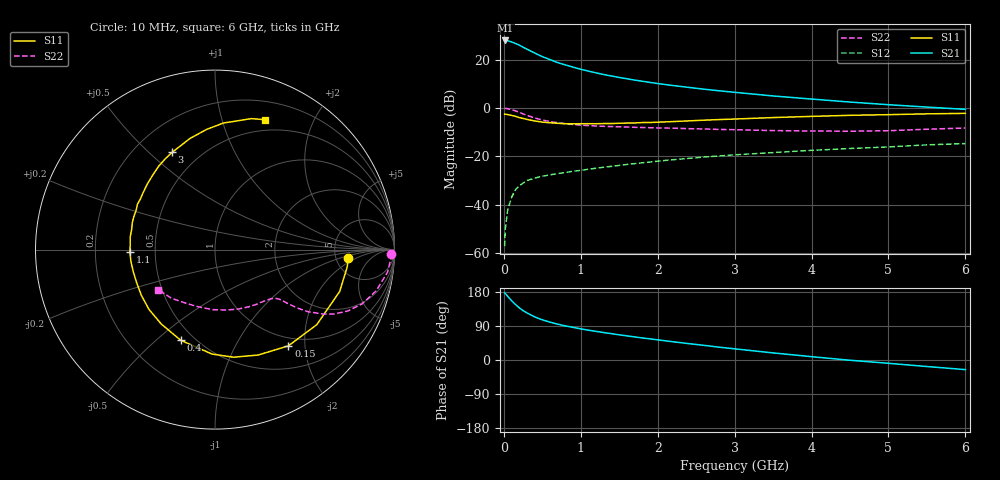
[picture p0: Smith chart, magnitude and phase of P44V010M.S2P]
! SIEMENS Small Signal Semiconductors
! BFP182
! Si NPN RF Bipolar Junction Transistor in SOT143
! VCE = 4 V  IC = 10 mA
! Common Emitter S-Parameters:  March  1996
# GHz  S  MA  R  50
!  f  S11  S21  S12  S22
! GHz  MAG  ANG  MAG  ANG  MAG  ANG  MAG  ANG
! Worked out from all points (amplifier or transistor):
!   36 points, 10 MHz to 6 GHz, reference 50 ohm
!   highest |S21| = 27.9 dB at 20 MHz (marker M1)
!   |S21| within 3 dB of that: start of sweep to 263.1 MHz
!   unconditionally stable (mu >= 1): 1.182 GHz to 5.382 GHz
!   at 250 MHz: K = 0.33, MSG = 28.1 dB, |S12| = -31.0 dB
!   at 1.4 GHz: K = 1.07, MAG = 17.1 dB, |S12| = -24.1 dB
!   at 6 GHz: K = 0.94, MSG = 7.1 dB, |S12| = -14.7 dB
!   lowest NFmin = 1.50 dB at 450 MHz
!   S11 on the Smith chart (normalised r, x): 10 MHz: 6.51, -1.40; 150 MHz: 0.86, -1.68; 400 MHz: 0.42, -0.60; 1.1 GHz: 0.36, -0.01; 3 GHz: 0.36, +0.59; 6 GHz: 0.38, +1.38
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0.01  0.7442 -3.7  24.84 177.5  0.0014 91.8  0.9828 -1.4
0.02  0.743 -7.5  24.86 175.4  0.0033 84.0  0.9813 -2.9
0.05  0.7327 -18.6  24.54 168.0  0.0078 83.6  0.9692 -7.5
0.1  0.7047 -36.4  23.18 156.8  0.0142 71.0  0.9265 -14.4
0.15  0.6743 -52.7  21.58 146.7  0.0204 65.5  0.8743 -20.2
0.2  0.6348 -67.7  19.93 137.7  0.0247 60.7  0.8151 -24.8
0.25  0.6084 -80.2  18.04 130.3  0.0281 56.0  0.7567 -28.3
0.3  0.5823 -91.6  16.41 124.4  0.0317 53.2  0.7064 -30.6
0.4  0.54 -110.7  13.69 113.8  0.0356 48.8  0.6245 -33.7
0.5  0.5114 -125.8  11.52 106.0  0.0389 45.5  0.5647 -35.3
0.6  0.4963 -137.9  9.987 99.9  0.0417 44.8  0.5241 -36.1
0.7  0.4828 -148.3  8.676 94.6  0.0441 44.2  0.4955 -36.7
0.9  0.4716 -164.7  6.98 86.1  0.0494 44.5  0.4565 -37.5
1.1  0.4744 -178.2  5.785 78.6  0.0544 44.4  0.4333 -38.9
1.5  0.4843 162.2  4.275 66.4  0.0652 44.5  0.4093 -42.8
1.8  0.5008 149.7  3.572 58.2  0.0739 44.5  0.3957 -46.6
2.2  0.5245 136.1  2.913 48.1  0.0856 42.8  0.3829 -52.8
3  0.592 113.8  2.11 29.5  0.108 38.2  0.3565 -68.4
3.5  0.6348 102.7  1.774 18.7  0.1201 34.6  0.3421 -79.7
4.5  0.7068 86.2  1.328 -0.7  0.1457 27.3  0.3319 -105.7
5.5  0.7573 74.5  1.045 -17.2  0.1733 20.2  0.3643 -132.1
6  0.7753 69.0  0.939 -25.4  0.1844 15.5  0.3868 -144.7
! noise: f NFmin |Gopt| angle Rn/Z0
0.45  1.5  0.26  43  0.28
0.9  1.6  0.24  87  0.22
1.8  2.1  0.2  170  0.2
